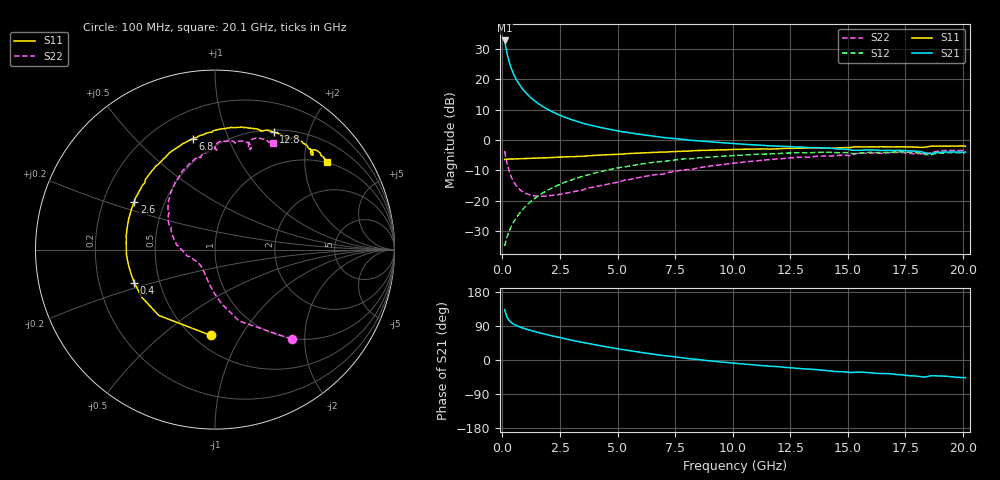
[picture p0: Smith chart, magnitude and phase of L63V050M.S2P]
!  Infineon Technologies AG
! BFR380L3 , PF131585-7, No.6, Th 09.10.01, soldered on pcb-board, measured with PP GSG850
!  Vce=3.0 V,  Ic=50.0 mA
! Common Emitter S-Parameters:  15. November 2001
#  GHz  S  MA  R  50
! f  S11  S21  S12  S22
! GHz  Mag  Ang  Mag  Ang  Mag  Ang  Mag  Ang
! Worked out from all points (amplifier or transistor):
!   201 points, 100 MHz to 20.1 GHz, reference 50 ohm
!   highest |S21| = 32.8 dB at 100 MHz (marker M1)
!   |S21| within 3 dB of that: start of sweep to 173.5 MHz
!   unconditionally stable (mu >= 1): 947.2 MHz to 4.182 GHz
!   at 3.4 GHz: K = 1.02, MAG = 8.2 dB, |S12| = -12.1 dB
!   at 10.1 GHz: K = 0.95, MSG = 1.9 dB, |S12| = -5.1 dB
!   at 20.1 GHz: K = 0.99, MSG = 0.1 dB, |S12| = -4.1 dB
!   S11 on the Smith chart (normalised r, x): 100 MHz: 0.60, -0.75; 400 MHz: 0.36, -0.17; 2.6 GHz: 0.33, +0.25; 6.8 GHz: 0.37, +0.75; 12.8 GHz: 0.53, +1.49; 20.1 GHz: 0.99, +2.57
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0.1  0.4783 -92.9  43.52 132.9  0.01786 62.9  0.6566 -49.4
0.2  0.4824 -130.5  27.2 113.3  0.02516 57.7  0.4196 -71.4
0.3  0.4868 -147.2  19.23 104.2  0.03173 60.7  0.3044 -83.0
0.4  0.4862 -157.6  14.77 98.5  0.03849 63.1  0.2412 -91.2
0.5  0.487 -164.1  11.95 94.4  0.04507 64.8  0.2031 -97.6
0.6  0.4891 -169.3  10.02 91.3  0.05192 66.6  0.178 -103.0
0.7  0.4917 -173.4  8.647 88.7  0.05871 67.7  0.1605 -107.9
0.8  0.4939 -176.8  7.599 86.2  0.06597 68.4  0.1481 -112.0
0.9  0.4941 -179.4  6.771 84.1  0.07297 68.8  0.139 -115.8
1  0.4948 177.8  6.117 82.2  0.08009 69.1  0.1327 -119.4
1.3  0.5008 171.1  4.743 76.8  0.1015 69.0  0.1221 -128.4
1.6  0.505 165.2  3.884 71.9  0.1232 68.1  0.1189 -135.7
2  0.5114 158.4  3.144 65.9  0.1514 66.3  0.1207 -143.8
2.6  0.523 149.3  2.466 57.7  0.1932 62.8  0.13 -154.0
3.5  0.5393 136.8  1.889 46.2  0.2539 56.7  0.1498 -165.5
5.1  0.583 118.4  1.393 28.5  0.3527 45.2  0.2046 174.2
6.8  0.6299 101.4  1.124 13.2  0.4398 33.2  0.2723 154.0
10.1  0.6991 77.3  0.868 -8.6  0.5574 11.4  0.4181 124.4
12.8  0.7326 63.4  0.768 -22.1  0.6158 -5.3  0.5182 102.4
13.5  0.7357 60.2  0.7484 -24.9  0.6212 -9.2  0.5304 98.0
16.8  0.7691 47.7  0.6738 -36.0  0.6271 -25.1  0.6186 77.4
20.1  0.7911 38.0  0.6329 -46.5  0.6203 -38.7  0.6751 61.5
